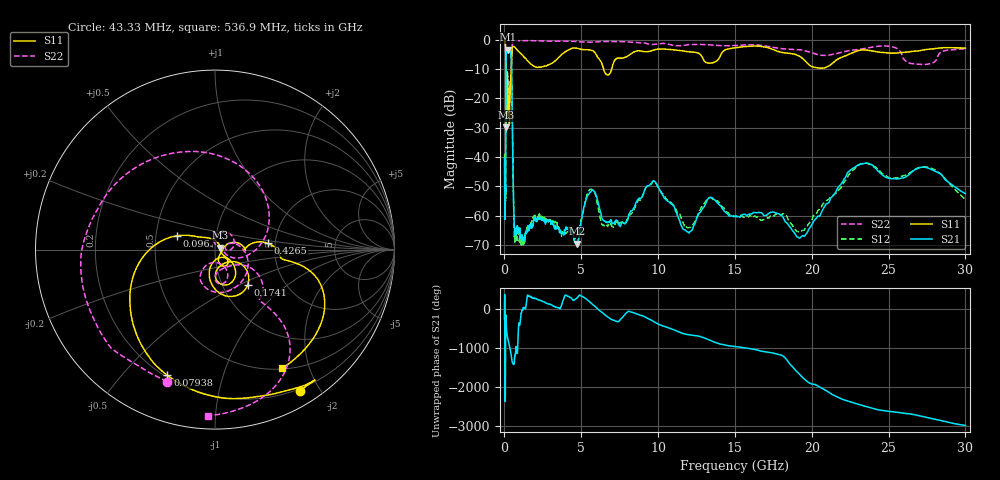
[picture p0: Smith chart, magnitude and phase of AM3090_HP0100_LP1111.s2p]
! Date/Time: Thu, Feb 28, 2019 1:58 PM
! Network Analyzer: Agilent Technologies E8364B Rev: A.07.50.67
! Sweep from 0.010 to 30.000 GHz, 1601 Points, Sweep Type: LOG
! Power Supply: 5.023 V, 0.002 A
# Hz S DB R 50
!freq MagS11 AngS11 MagS21 AngS21 MagS12 AngS12 MagS22 AngS22
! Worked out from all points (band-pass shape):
!   1601 points, 10 MHz to 30 GHz, reference 50 ohm
!   highest |S21| = -3.32 dB at 262.5 MHz (marker M1); lowest = -69.6 dB at 4.734 GHz (marker M2)
!   |S21| within 3 dB of the highest: 108.2 MHz to 441.6 MHz (333.4 MHz wide, 121 % of centre)
!   lowest |S11| = -29.8 dB at 103.5 MHz (marker M3), VSWR 1.07, Z = 53.1 + j1.18 ohm
!   |S11| at or under -10 dB: 94.47 MHz to 429.8 MHz (335.3 MHz wide, 128 % of centre); 6.454 GHz to 6.978 GHz (524.4 MHz wide, 7.81 % of centre)
!   |S22| runs from -31.9 to -0.2 dB; largest |S21 - S12| = 0.012
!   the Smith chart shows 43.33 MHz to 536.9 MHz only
!   S11 on the Smith chart (normalised r, x): 43.33 MHz: 0.18, -1.76; 79.38 MHz: 0.21, -0.67; 96 MHz: 0.64, +0.10; 174.1 MHz: 1.31, -0.56; 426.5 MHz: 1.83, +0.14; 536.9 MHz: 0.51, -1.59
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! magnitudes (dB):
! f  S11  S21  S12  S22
! 10 MHz  -0.3  -40.4  -38.9  -0.7
! 38.04 MHz  -0.5  -60.1  -59.1  -1.7
! 43.33 MHz  -0.8  -60.1  -60.4  -2.1
! 79.38 MHz  -2.5  -50.1  -47.8  -4.5
! 96 MHz  -12.9  -14.7  -14.8  -13.7
! 103.5 MHz  -29.8  -7.8  -7.8  -31.7
! 144.7 MHz  -20.5  -3.8  -3.7  -24.7
! 174.1 MHz  -11.4  -3.5  -3.5  -14.1
! 262.5 MHz  -22.5  -3.3  -3.3  -17.2
! 426.5 MHz  -10.5  -5.4  -5.4  -10.6
! 536.9 MHz  -2.4  -38.1  -38.0  -0.7
! 550.5 MHz  -2.3  -42.9  -42.8  -0.5
! 659.1 MHz  -2.5  -64.5  -67.3  -0.2
! 2.084 GHz  -9.4  -62.1  -62.0  -0.3
! 4.734 GHz  -2.9  -69.6  -66.8  -0.6
! 5.64 GHz  -3.5  -51.7  -51.0  -0.8
! 7.926 GHz  -5.8  -62.4  -62.2  -0.7
! 9.634 GHz  -3.6  -48.3  -48.6  -1.6
! 11.83 GHz  -4.0  -65.2  -63.8  -1.8
! 19.31 GHz  -6.0  -67.2  -65.4  -3.4
! 23.48 GHz  -3.4  -42.2  -42.2  -2.9
! 30 GHz  -2.8  -52.5  -54.6  -3.1
